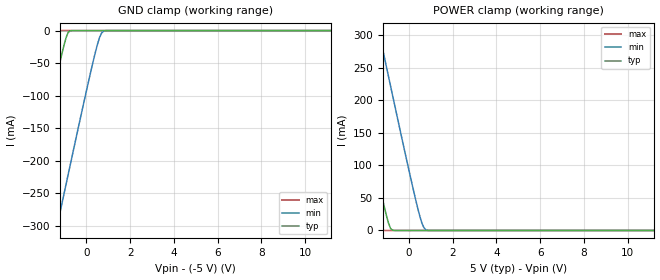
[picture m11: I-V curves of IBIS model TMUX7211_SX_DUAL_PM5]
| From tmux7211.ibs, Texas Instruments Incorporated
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[Model]   TMUX7211_SX_DUAL_PM5
Model_type   Terminator
|   typ   min   max
C_comp   0pF   0pF   0pF
[Voltage Range]   10   10   10
[Temperature Range]   27   130   -40
[Power Clamp Reference]   5   5   5
[GND Clamp Reference]   -5   -5   -5
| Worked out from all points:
|   GND clamp passes 1 mA (typ) near -0.77 V on its own axis
|   POWER clamp passes 1 mA (typ) near -0.77 V on its own axis
[GND Clamp]
|   Voltage   I(typ)   I(min)   I(max)
-30V      -4.646A    -4.881A    -4.408A
-4.44V    -555.4mA   -791.7mA   -317.7mA
-4.35V    -541mA     -777.4mA   -303.4mA
-2.91V    -312.6mA   -548.5mA   -77.36mA
-2.46V    -241.6mA   -477.2mA   -12.06mA
-2.28V    -213.3mA   -448.7mA   -147.7uA
-1.47V    -87.59mA   -320.9mA   0A
-1.29V    -60.46mA   -292.5mA   0A
-840mV    -3.269mA   -222.1mA   0A
420mV     0A         -32.2mA    0A
870mV     0A         -118.6uA   0A
60V       0A         0A         0A
[POWER Clamp]
|   Voltage   I(typ)   I(min)   I(max)
-30V      4.646A     4.881A     4.408A
-4.44V    555.4mA    791.7mA    317.7mA
-4.35V    541mA      777.4mA    303.4mA
-2.91V    312.6mA    548.5mA    77.36mA
-2.46V    241.6mA    477.2mA    12.06mA
-2.28V    213.3mA    448.7mA    147.7uA
-1.47V    87.59mA    320.9mA    0A
-1.29V    60.46mA    292.5mA    0A
-840mV    3.269mA    222.1mA    0A
420mV     0A         32.2mA     0A
870mV     0A         118.6uA    0A
60V       0A         0A         0A
